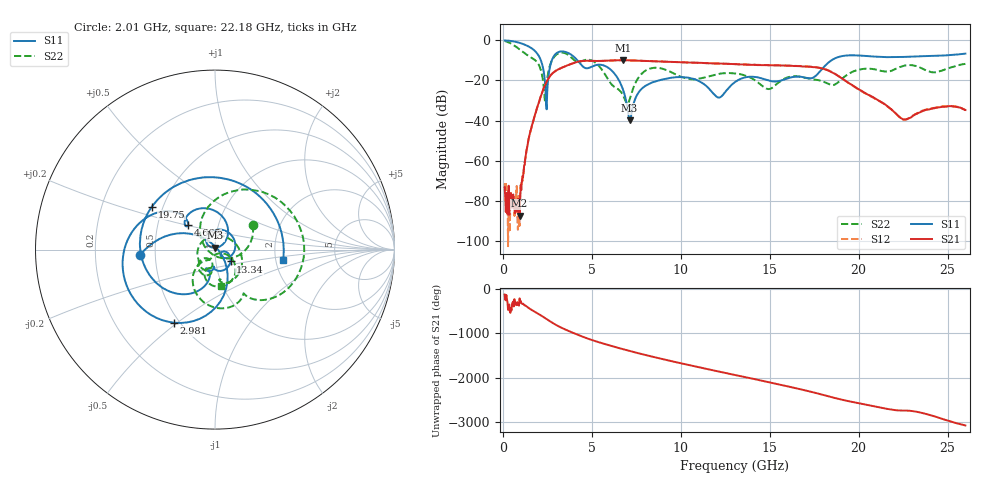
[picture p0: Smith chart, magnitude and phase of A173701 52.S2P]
!  2-Port S-parameters saved by WinCal
! VAR MeasName=S-Parameters (CALIBRATED_DATA) read from VNA (N5245A)
! VAR MeasDate=2017-6-7 10:31:52
! VAR NAME=A173701 52
! VAR FILENAME=A173701 52.S2P
! VAR DATE=2017-6-7 10:31:52
! VAR PHYS_PORTS=1,2
# Hz S DB R 50
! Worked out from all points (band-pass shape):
!   801 points, 100 MHz to 26 GHz, reference 50 ohm
!   highest |S21| = -9.87 dB at 6.737 GHz (marker M1); lowest = -87.5 dB at 941.8 MHz (marker M2)
!   |S21| within 3 dB of the highest: 3.517 GHz to 16.74 GHz (13.22 GHz wide, 131 % of centre)
!   lowest |S11| = -39.9 dB at 7.125 GHz (marker M3), VSWR 1.02, Z = 50.1 + j1.01 ohm
!   |S11| at or under -10 dB: 2.14 GHz to 2.752 GHz (611.2 MHz wide, 25 % of centre); 4.198 GHz to 18.46 GHz (14.26 GHz wide, 126 % of centre)
!   |S22| runs from -31.7 to -0.2 dB; largest |S21 - S12| = 0.0038
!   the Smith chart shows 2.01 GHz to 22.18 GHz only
!   S11 on the Smith chart (normalised r, x): 2.01 GHz: 0.41, -0.03; 2.981 GHz: 0.47, -0.49; 4.665 GHz: 0.71, +0.20; 13.34 GHz: 1.18, -0.16; 19.75 GHz: 0.44, +0.25; 22.18 GHz: 2.20, -0.30
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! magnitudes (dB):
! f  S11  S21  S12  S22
! 100 MHz  0.0  -73.4  -71.4  -0.2
! 941.8 MHz  -1.2  -87.5  -92.6  -4.5
! 1.46 GHz  -3.1  -48.8  -48.7  -7.8
! 2.01 GHz  -7.6  -31.3  -31.3  -12.0
! 2.463 GHz  -34.4  -20.6  -20.6  -21.3
! 2.981 GHz  -6.6  -15.1  -15.1  -7.3
! 4.438 GHz  -12.5  -10.3  -10.3  -10.3
! 4.665 GHz  -13.9  -10.2  -10.2  -9.7
! 5.863 GHz  -13.3  -10.1  -10.2  -18.7
! 6.737 GHz  -24.1  -9.9  -9.9  -27.0
! 7.125 GHz  -39.9  -10.0  -9.9  -29.5
! 7.773 GHz  -24.4  -10.2  -10.2  -16.9
! 8.744 GHz  -20.0  -10.5  -10.5  -13.7
! 12.14 GHz  -28.5  -11.5  -11.5  -16.7
! 13.05 GHz  -20.8  -11.8  -11.8  -16.5
! 13.34 GHz  -19.3  -12.0  -11.9  -16.9
! 14.93 GHz  -20.0  -12.4  -12.3  -24.3
! 17.39 GHz  -18.7  -13.3  -13.2  -19.4
! 19.75 GHz  -7.4  -23.0  -23.1  -15.3
! 21.69 GHz  -8.3  -33.4  -33.5  -15.5
! 22.18 GHz  -8.3  -37.3  -37.3  -13.8
! 26 GHz  -6.6  -34.8  -34.7  -11.7
